FUNCTION_BLOCK FB_NcBasedHoming
VAR_IN_OUT
	AxisRef	: AXIS_REF;
END_VAR
VAR_INPUT
	bExcute		: BOOL;
	bReset		: BOOL;
	stParameter	: ST_Parameter_HomeConfig;
END_VAR
VAR_OUTPUT
	bHoming			: BOOL;
	bBiasWriting	: BOOL;
	bBlockHoming	: BOOL;
	bError			: BOOL;
	nErrorID		: UDINT;
	eHomeStep		: E_NCHomeStep;
END_VAR
VAR
	fbHome 					: MC_Home; 					(* Function Block*)
	fbHomeAbsoluteSwitch	: MC_StepAbsoluteSwitch; 	(* Function Block*)
	fbHomeLimitSwitch		: MC_StepLimitSwitch;		(* Function Block*)
	fbHomeZpulse			: MC_StepReferencePulse;	(* Function Block*)
	fbFinishHome			: MC_FinishHoming; 			(* Function Block*)
	fbSetPosition			: MC_SetPosition; 			(* Function Block*)
	fbStepBlockLagBased		: MC_StepBlockLagBased; 	(* Function Block*)
	fbAbortHoming			: MC_AbortHoming; 			(* Function Block*)
	fbAdsWrite				: ADSWRITE;                 (* Function Block*)
	fbCoEWrite1				: FB_CoEWrite;
	fbCoEWrite2				: FB_CoEWrite;
	HomeParameter			: MC_HomingParameter;		(* 回零参数，不需要更改*)		
	fPositionBias			: LREAL;
	ZERO_HOME_OFFSET		: LREAL := 0;
	rtExecute: R_TRIG;
	rtAbort: R_TRIG;
	BlockHomeHwTorqueLimit: UINT;
	old_NcCycleCounter: UDINT;
END_VAR

rtExecute( CLK := bExcute );
rtAbort	( CLK := bReset );


IF rtExecute.Q THEN
	fbHome.Execute 					:= FALSE;
	fbHomeAbsoluteSwitch.Execute 	:= FALSE;
	fbHomeLimitSwitch.Execute 		:= FALSE;
	fbHomeZpulse.Execute 			:= FALSE;
	fbStepBlockLagBased.Execute		:= FALSE;
	fbFinishHome.Execute 			:= FALSE;
	fbSetPosition.Execute			:= FALSE;
	nErrorID	:= 0;
	CASE stParameter.HomeMode OF
		ABSOLUTESWITCH 	:
			eHomeStep := STATE_HOME_DISABLELIMIT;
	    LIMITSWITCH 	:
			eHomeStep := STATE_HOME_DISABLELIMIT;
	    DIRECTHOME		:
			eHomeStep := STATE_HOME_ADS_RESET;
	    ZPULSEHOME		:
			eHomeStep := STATE_HOME_ZPULSE;
	    SETPOSITION		:
			eHomeStep := STATE_CLEAR_POSITION;
	    BLOCKHOME		:
			eHomeStep := STATE_HOME_DISABLELIMIT;
	END_CASE
ELSIF rtAbort.Q THEN
	fbAbortHoming.Execute			:= FALSE;
	eHomeStep := STATE_HOME_ABORTING;
ELSIF bExcute = FALSE AND bReset = FALSE THEN
	fbHome.Execute 					:= FALSE;
	fbHomeAbsoluteSwitch.Execute 	:= FALSE;
	fbHomeLimitSwitch.Execute 		:= FALSE;
	fbHomeZpulse.Execute 			:= FALSE;
	fbStepBlockLagBased.Execute		:= FALSE;
	fbAbortHoming.Execute			:= FALSE;
	fbFinishHome.Execute 			:= FALSE;
	fbSetPosition.Execute			:= FALSE;
	eHomeStep := STATE_HOME_STANDSTILL;
END_IF

bBiasWriting 	:= FALSE;
bBlockHoming 	:= FALSE;
bHoming			:= FALSE;
bError			:= eHomeStep = STATE_HOME_ERROR;
IF eHomeStep <> STATE_HOME_STANDSTILL AND eHomeStep <> STATE_HOME_DONE AND eHomeStep <> STATE_HOME_ERROR THEN
	bHoming		:= TRUE;
END_IF
IF eHomeStep >= STATE_HOME_ADS_RESET AND eHomeStep <= STATE_HOME_ADS_FINISH THEN
	bBiasWriting := TRUE;
ELSIF eHomeStep >= STATE_HOME_BLOCK_1 AND eHomeStep <= STATE_HOME_BLOCK_3 THEN
	bBlockHoming := TRUE;
END_IF

CASE eHomeStep OF
(**********************HOME DIRECT****************************)
STATE_HOME_ADS_RESET:
	fbHome.HomingMode		:= MC_HomingMode.MC_ResetCalibration;
	fbHome.Execute			:= TRUE;
	IF fbHome.Done THEN
		fbHome.Execute		:= FALSE;
		eHomeStep 			:= STATE_HOME_ADS1;
	ELSIF fbHome.Error THEN
		fbHome.Execute		:= FALSE;
		eHomeStep 			:= STATE_HOME_ERROR;
	END_IF

STATE_HOME_ADS1:
	fPositionBias			:= stParameter.HomeOffset;
	fbAdsWrite.SRCADDR		:= ADR(fPositionBias);
	fbAdsWrite.WRITE		:= TRUE;
	IF fbAdsWrite.BUSY THEN
		fbAdsWrite.WRITE	:= FALSE;
		eHomeStep 			:= STATE_HOME_ADS2;
	END_IF	
	
STATE_HOME_ADS2:
	IF (NOT fbAdsWrite.BUSY) AND (NOT fbAdsWrite.ERR) THEN
		eHomeStep 		:= STATE_HOME_ADS_FINISH;
	ELSIF fbAdsWrite.ERR THEN
		fbAdsWrite.WRITE		:= FALSE;
		eHomeStep				:= STATE_HOME_ERROR;
		nErrorID := fbAdsWrite.ERRID;
	END_IF
	
STATE_HOME_ADS_FINISH:
	fbHome.HomingMode		:= MC_HomingMode.MC_ForceCalibration;
	fbHome.Execute			:= TRUE;
	IF fbHome.Done THEN
		fbHome.Execute		:= FALSE;
		eHomeStep 			:= STATE_HOME_DONE;
	ELSIF fbHome.Error THEN
		fbHome.Execute		:= FALSE;
		eHomeStep 			:= STATE_HOME_ERROR;
	END_IF
	
	
(******************** HOME DISABLE LIMIT**********************)
STATE_HOME_DISABLELIMIT:
	MC_SetAcceptBlockedDriveSignal(Axis := AxisRef,Enable := TRUE);
	fbHome.HomingMode		:= MC_HomingMode.MC_ResetCalibration;
	fbHome.Execute			:= TRUE;
	IF fbHome.Done THEN
		fbHome.Execute		:= FALSE;
		IF stParameter.HomeMode = E_HomeMode.ABSOLUTESWITCH THEN
			eHomeStep := STATE_HOME_ABSOLUTESWITCH;
		ELSIF stParameter.HomeMode = E_HomeMode.LIMITSWITCH THEN
			eHomeStep := STATE_HOME_LIMITSWITCH;
		ELSIF stParameter.HomeMode = E_HomeMode.BLOCKHOME THEN
			eHomeStep := STATE_HOME_BLOCK_1;
		END_IF
		
	ELSIF fbHome.Error THEN
		fbHome.Execute		:= FALSE;
		eHomeStep 			:= STATE_HOME_ERROR;
		
	END_IF
	
(******************** HOME ABSOLUTE SWITCH**********************)
STATE_HOME_ABSOLUTESWITCH: (* STATE: start homing process *)
	
	fbHomeAbsoluteSwitch.Direction 		:= stParameter.StartDirection;
	fbHomeAbsoluteSwitch.SwitchMode 	:= stParameter.SwitchMode;
	fbHomeAbsoluteSwitch.Velocity 		:= stParameter.HomeVelocity;
	fbHomeAbsoluteSwitch.SetPosition	:= stParameter.HomeOffset;
	fbHomeAbsoluteSwitch.Execute		:= TRUE;
	
	IF (fbHomeAbsoluteSwitch.Done = TRUE) THEN
		fbHomeAbsoluteSwitch.Execute := FALSE;
		IF stParameter.EnableZpulseHome THEN
			eHomeStep := STATE_HOME_ZPULSE;
		ELSE
			eHomeStep := STATE_HOME_FINISH;
		END_IF
	END_IF
	(* if a homing error occured go to error state *)
	IF (fbHomeAbsoluteSwitch.Error = TRUE) THEN
		fbHomeAbsoluteSwitch.Execute := FALSE;
		nErrorID := fbHomeAbsoluteSwitch.ErrorID;
		eHomeStep := STATE_HOME_ERROR;
	END_IF


(******************** HOME LIMIT SWITCH**********************)
STATE_HOME_LIMITSWITCH:
	fbHomeLimitSwitch.Direction 		:= stParameter.StartDirection;
	fbHomeLimitSwitch.LimitSwitchMode 	:= stParameter.SwitchMode;
	fbHomeLimitSwitch.Velocity 			:= stParameter.HomeVelocity;
	fbHomeLimitSwitch.SetPosition 		:= stParameter.HomeOffset;
	fbHomeLimitSwitch.Execute			:= TRUE;
	AxisRef.ReadStatus();
	IF (fbHomeLimitSwitch.Done = TRUE)AND (AxisRef.Status.NotMoving) THEN
		fbHomeLimitSwitch.Execute := FALSE;
		IF stParameter.EnableZpulseHome THEN
			eHomeStep := STATE_HOME_ZPULSE;
		ELSE
			eHomeStep := STATE_HOME_FINISH;
		END_IF
	END_IF
	(* if a homing error occured go to error state *)
	IF (fbHomeLimitSwitch.Error = TRUE) THEN
		fbHomeLimitSwitch.Execute := FALSE;
		nErrorID := fbHomeLimitSwitch.ErrorID;
		eHomeStep := STATE_HOME_ERROR;
	END_IF

(******************** HOME ZPulse**********************)
STATE_HOME_ZPULSE:
	fbHomeZpulse.SetPosition	:= stParameter.HomeOffset;//2023.4.18日，修改寻Z脉冲之后的设定位置为回零偏置。
	fbHomeZpulse.Velocity		:= stParameter.HomeZPulseVelocity;
	fbHomeZpulse.Execute			:= TRUE;
	AxisRef.ReadStatus();
	IF (fbHomeZpulse.Done = TRUE)AND (AxisRef.Status.NotMoving) THEN
		fbHomeZpulse.Execute := FALSE;
		eHomeStep := STATE_HOME_FINISH;
	END_IF
	(* if a homing error occured go to error state *)
	IF (fbHomeZpulse.Error = TRUE) THEN
		fbHomeZpulse.Execute := FALSE;
		nErrorID := fbHomeZpulse.ErrorID;
		eHomeStep := STATE_HOME_ERROR;
	END_IF

(******************** HOME BLOCK**********************)	
STATE_HOME_BLOCK_1:
	BlockHomeHwTorqueLimit := LREAL_TO_UINT(stParameter.BlockHomeTorqueLimit) * 10;
	
	fbCoEWrite1.Index		:= 16#60E0;
	fbCoEWrite1.SubIndex		:= 0;
	fbCoEWrite1.pSrcBuf		:= ADR( BlockHomeHwTorqueLimit );
	fbCoEWrite1.BufLen		:= SIZEOF( BlockHomeHwTorqueLimit );
	fbCoEWrite1( Axis := AxisRef , Execute := TRUE );
	
	fbCoEWrite2.Index		:= 16#60E1;
	fbCoEWrite2.SubIndex		:= 0;
	fbCoEWrite2.pSrcBuf		:= ADR( BlockHomeHwTorqueLimit );
	fbCoEWrite2.BufLen		:= SIZEOF( BlockHomeHwTorqueLimit );
	fbCoEWrite2( Axis := AxisRef , Execute := TRUE );
	
	IF fbCoEWrite1.Busy = FALSE AND fbCoEWrite2.Busy = FALSE THEN
		IF fbCoEWrite1.Error = FALSE AND fbCoEWrite2.Error = FALSE THEN
			fbCoEWrite1( Axis := AxisRef , Execute := FALSE );
			fbCoEWrite2( Axis := AxisRef , Execute := FALSE );
			eHomeStep := STATE_HOME_BLOCK_2;
		ELSE
			fbCoEWrite1( Axis := AxisRef , Execute := FALSE );
			fbCoEWrite2( Axis := AxisRef , Execute := FALSE );
			nErrorID := fbCoEWrite1.CANopenErrId OR fbCoEWrite2.CANopenErrId ;
			eHomeStep := STATE_HOME_ERROR;
		END_IF
	END_IF
	
//BlockHomeHwTorqueLimit := 3000;
STATE_HOME_BLOCK_2:
	fbStepBlockLagBased.Direction 		:= stParameter.StartDirection;
	fbStepBlockLagBased.Velocity		:= stParameter.HomeVelocity;
	fbStepBlockLagBased.Acceleration	:= stParameter.Acceleration;
	fbStepBlockLagBased.Deceleration	:= stParameter.Deceleration;
	fbStepBlockLagBased.Jerk			:= stParameter.Jerk;
	fbStepBlockLagBased.SetPosition		:= stParameter.HomeOffset;
	fbStepBlockLagBased.DetectionVelocityLimit		:= stParameter.BlockHomeDetectionVeloLimit;
	fbStepBlockLagBased.DetectionVelocityTime		:= stParameter.BlockHomeDetectionVeloTime;
	fbStepBlockLagBased.TimeLimit		:= stParameter.BlockHomeTimeLimit;
	fbStepBlockLagBased.DistanceLimit	:= stParameter.BlockHomeDistanceLimit;
	fbStepBlockLagBased.TorqueLimit		:= stParameter.BlockHomeTorqueLimit;
	fbStepBlockLagBased.LagLimit		:= stParameter.BlockHomeLagLimit;
	fbStepBlockLagBased.Execute			:= TRUE;
	AxisRef.ReadStatus();
	IF (fbStepBlockLagBased.Done = TRUE)AND (AxisRef.Status.NotMoving) THEN
		fbStepBlockLagBased.Execute := FALSE;
		eHomeStep := STATE_HOME_BLOCK_3;
	END_IF
	(* if a homing error occured go to error state *)
	IF (fbStepBlockLagBased.Error = TRUE) THEN
		fbStepBlockLagBased.Execute := FALSE;
		nErrorID := fbStepBlockLagBased.ErrorID;
		eHomeStep := STATE_HOME_ERROR;
	END_IF
	
STATE_HOME_BLOCK_3:
	BlockHomeHwTorqueLimit := 3000;
	
	fbCoEWrite1.Index		:= 16#60E0;
	fbCoEWrite1.SubIndex		:= 0;
	fbCoEWrite1.pSrcBuf		:= ADR( BlockHomeHwTorqueLimit );
	fbCoEWrite1.BufLen		:= SIZEOF( BlockHomeHwTorqueLimit );
	fbCoEWrite1( Axis := AxisRef , Execute := TRUE );
	
	fbCoEWrite2.Index		:= 16#60E1;
	fbCoEWrite2.SubIndex		:= 0;
	fbCoEWrite2.pSrcBuf		:= ADR( BlockHomeHwTorqueLimit );
	fbCoEWrite2.BufLen		:= SIZEOF( BlockHomeHwTorqueLimit );
	fbCoEWrite2( Axis := AxisRef , Execute := TRUE );
	
	IF fbCoEWrite1.Busy = FALSE AND fbCoEWrite2.Busy = FALSE THEN
		fbCoEWrite1( Axis := AxisRef , Execute := FALSE );
		fbCoEWrite2( Axis := AxisRef , Execute := FALSE );
		IF fbCoEWrite1.Error = FALSE AND fbCoEWrite2.Error = FALSE THEN
			IF stParameter.EnableZpulseHome THEN
				eHomeStep := STATE_HOME_ZPULSE;
			ELSE
				eHomeStep := STATE_HOME_FINISH;
			END_IF
		ELSE
			nErrorID := fbCoEWrite1.CANopenErrId OR fbCoEWrite2.CANopenErrId ;
			eHomeStep := STATE_HOME_ERROR;
		END_IF
	END_IF	
(********************Aborting Home**********************)	
STATE_HOME_ABORTING:	

	BlockHomeHwTorqueLimit := 3000;
	
	fbCoEWrite1.Index		:= 16#60E0;
	fbCoEWrite1.SubIndex		:= 0;
	fbCoEWrite1.pSrcBuf		:= ADR( BlockHomeHwTorqueLimit );
	fbCoEWrite1.BufLen		:= SIZEOF( BlockHomeHwTorqueLimit );
	fbCoEWrite1( Axis := AxisRef , Execute := TRUE );
	
	fbCoEWrite2.Index		:= 16#60E1;
	fbCoEWrite2.SubIndex		:= 0;
	fbCoEWrite2.pSrcBuf		:= ADR( BlockHomeHwTorqueLimit );
	fbCoEWrite2.BufLen		:= SIZEOF( BlockHomeHwTorqueLimit );
	fbCoEWrite2( Axis := AxisRef , Execute := TRUE );
	
	fbAbortHoming.Execute := TRUE;
	
	IF fbCoEWrite1.Busy = FALSE AND fbCoEWrite2.Busy = FALSE AND (fbAbortHoming.Done = TRUE) THEN
		fbCoEWrite1( Axis := AxisRef , Execute := FALSE );
		fbCoEWrite2( Axis := AxisRef , Execute := FALSE );
		IF fbCoEWrite1.Error = FALSE AND fbCoEWrite2.Error = FALSE THEN
			IF nErrorID = 0 THEN
				eHomeStep := STATE_HOME_DONE;
			ELSE
				eHomeStep := STATE_HOME_ERROR;
			END_IF
		ELSE
			nErrorID := fbCoEWrite1.CANopenErrId OR fbCoEWrite2.CANopenErrId ;
			eHomeStep := STATE_HOME_ERROR;
		END_IF
	END_IF	

	(* if a homing error occured go to error state *)
	IF (fbAbortHoming.Error = TRUE) THEN
		fbAbortHoming.Execute := FALSE;
		nErrorID := fbAbortHoming.ErrorID;
		eHomeStep := STATE_HOME_ERROR;
	END_IF
	
	
(********************FINISH HOME**********************)	
STATE_HOME_FINISH:
	fbFinishHome.Velocity := stParameter.HomeVelocityCorrect;
	fbFinishHome.Distance :=  - AxisRef.NcToPlc.SetPos;//stParameter.HomeOffset  2023.4.18日，修改  2023.8.29再次修改
	fbFinishHome.Execute		:= TRUE;
	IF (fbFinishHome.Done = TRUE) THEN
		fbFinishHome.Execute := FALSE;
		eHomeStep := STATE_HOME_ENABLELIMIT;
	END_IF
	(* if a homing error occured go to error state *)
	IF (fbFinishHome.Error = TRUE) THEN
		fbFinishHome.Execute := FALSE;
		nErrorID := fbFinishHome.ErrorID;
		eHomeStep := STATE_HOME_ERROR;
	END_IF

(********************HOME ENABLE LIMIT**********************)		
STATE_HOME_ENABLELIMIT:
	MC_SetAcceptBlockedDriveSignal(Axis := AxisRef, Enable := FALSE);
	eHomeStep := STATE_HOME_DONE;


STATE_CLEAR_POSITION:
	fbSetPosition.Position := stParameter.HomeOffset;
	fbSetPosition.Execute := TRUE;
	IF (fbSetPosition.Done = TRUE) THEN
		fbSetPosition.Execute := FALSE;
		eHomeStep := STATE_CLEAR_POSITION_1;        
	END_IF
	(* check if error occured *)
	IF (fbSetPosition.Error = TRUE) THEN
		nErrorID := fbSetPosition.ErrorID;
		fbSetPosition.Execute := FALSE;
		eHomeStep := STATE_HOME_ERROR;
	END_IF 
	
STATE_CLEAR_POSITION_1:

	fbHome.HomingMode		:= MC_HomingMode.MC_ForceCalibration;
	fbHome.Execute			:= TRUE;
	IF fbHome.Done THEN
		fbHome.Execute		:= FALSE;
		eHomeStep 			:= STATE_HOME_DONE;
	ELSIF fbHome.Error THEN
		fbHome.Execute		:= FALSE;
		nErrorID := fbHome.ErrorID;
		eHomeStep 			:= STATE_HOME_ERROR;
	END_IF
	
END_CASE	







(************************** SET /RESET HOME CALIBRATION ****************************)
fbHome(Axis := AxisRef);

fbSetPosition( Axis:= AxisRef );

(************************** HOME ABSOLUTE SWITCH ****************************)
fbHomeAbsoluteSwitch.ReferenceSignal.Level 			:= stParameter.RefrenceSignal;
fbHomeAbsoluteSwitch.PositiveLimitSwitch 			:= stParameter.PositiveSwitch;
fbHomeAbsoluteSwitch.NegativeLimitSwitch 			:= stParameter.NegativeSwitch;
fbHomeAbsoluteSwitch.Options.DisableDriveAccess 	:= TRUE;
fbHomeAbsoluteSwitch(Axis := AxisRef,Parameter 		:= HomeParameter);
(************************** HOME LIMIT SWITCH ****************************)
IF fbHomeLimitSwitch.Direction = mcNegativeDirection THEN
	fbHomeLimitSwitch.LimitSwitchSignal.Level 		:= stParameter.NegativeSwitch;
ELSIF fbHomeLimitSwitch.Direction = mcPositiveDirection THEN
	fbHomeLimitSwitch.LimitSwitchSignal.Level 		:= stParameter.PositiveSwitch;
END_IF
fbHomeLimitSwitch.Options.DisableDriveAccess 		:= TRUE;
fbHomeLimitSwitch(Axis := AxisRef,Parameter 		:= HomeParameter);
(************************** HOME Zpulse SWITCH ****************************)
fbHomeZpulse.Direction								:= stParameter.ZPulseDirection;
fbHomeZpulse.ReferenceSignal.SignalSource			:= E_SignalSource.SignalSource_ZeroPulse;
fbHomeZpulse.ReferenceSignal.TouchProbe				:= E_TouchProbe.TouchProbe1;
fbHomeZpulse.Options.DisableDriveAccess				:= TRUE;
fbHomeZpulse(Axis := AxisRef,Parameter 	:= HomeParameter);
(************************** HOME BLOCK ****************************)

fbStepBlockLagBased.Options.DisableDriveAccess				:= TRUE;
fbStepBlockLagBased(Axis := AxisRef,Parameter 	:= HomeParameter);
(************************** HOME Aborting ****************************)
fbAbortHoming.Options.DisableDriveAccess := TRUE;
fbAbortHoming( Axis := AxisRef,Parameter 	:= HomeParameter );
(************************** FINISH HOME & SET FLAG ****************************)
fbFinishHome.Options.DisableDriveAccess 			:= TRUE;
fbFinishHome(Axis := AxisRef,Parameter 	:= HomeParameter);

(************************** ADS WRITE ****************************)
fbAdsWrite.PORT		:= 501;
fbAdsWrite.IDXGRP 	:= AxisRef.NcToPlc.AxisId + 16#00005000;
fbAdsWrite.IDXOFFS 	:= 16#00000007;
fbAdsWrite.LEN 		:= 8;
fbAdsWrite();

END_FUNCTION_BLOCK
